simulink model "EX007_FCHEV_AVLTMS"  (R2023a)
settings: Solver=ode23tb  StartTime=0.0  StopTime=20e3  RelTol=1e-3
libraries: component_lib x76, slpidlib x7, simulink x1

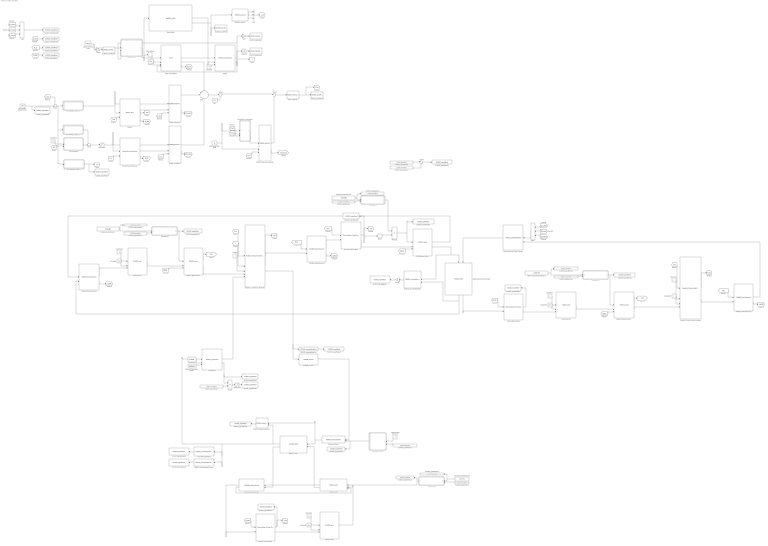
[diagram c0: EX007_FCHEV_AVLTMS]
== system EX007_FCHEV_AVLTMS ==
  Add : Sum  Inputs=+++
  Add1 : Sum  Inputs=+++
  Battery : component_lib/Battery Pack  SOC_0=0.5  Nx=120  Ny=180
  Battery Chiller : component_lib/Thermal Systems/RF0007_PHEX  N_ch=20  L=180e-3  B=65e-3  H=2e-3  t=0.3e-3  D_h=2.61e-3  N_nod=5
  Battery Thermal Mass : component_lib/Thermal Mass & Heat Transfer  n=100  d=10e-3  L=4  m=120 * 180 * 0.048  cp=1040  T_0=273 + 25
  Bus Voltage Control 1 : Subsystem
  "Bus Voltage Control 2 " : Subsystem
  Bus Voltage Control 3 : Subsystem
  Bus Voltage Reference [V] : Constant  Value=700
  Calculate Superheat1 : component_lib/Thermal Systems/RF0010_calculateSuperHeat
  Chassi : component_lib/Powertrain/PT0001_simpleVehicle  m=40e3  r_w=0.5  A_f=10  C_d=0.5  rho_air=1.225  c_r0=0.0060  c_r1=2.3e-7  gain=600  v0=75/3.6  x0=0
  Compressor : component_lib/Thermal Systems/RF0003_compressor  V_disp=0.00017  N_ref=2000
  Constant : Constant
  Constant1 : Constant  Value=0
  Constant10 : Constant
  Constant11 : Constant  Value=0
  Constant2 : Constant  Value=8
  Constant3 : Constant  Value=0.5
  Constant4 : Constant  Value=0.1
  Constant5 : Constant  Value=2e5
  Constant6 : Constant  Value=2e5
  Constant7 : Constant  Value=5
  Constant8 : Constant  Value=1.65e6
  Constant9 : Constant  Value=2e5
  Coolant Tank1 : component_lib/Thermal Systems/TH0013_tank  V=5e-3  T0=273.15 + 80
  Coolant Tank2 : component_lib/Thermal Systems/TH0013_tank  V=5e-3  T0=273.15 + 25
  Coolant Tank3 : component_lib/Thermal Systems/TH0013_tank  V=5e-3  T0=273.15 + 80
  DC/DC - Low level converter : component_lib/Electrochemistry/EL0008_dcdcConverter  eta_up=0.98  eta_down=0.98
  DC/DC Converter : component_lib/Electrochemistry/EL0008_dcdcConverter  eta_up=0.98  eta_down=0.98
  DC/DC Converter1 : component_lib/Electrochemistry/EL0008_dcdcConverter  eta_up=0.98  eta_down=0.98
  Divide : Product  Inputs=/*
  Expansion Valve : component_lib/Thermal Systems/RF0005_expansionValve  D=3*1.8e-3  p_min=100e3
  Fuel Cell Thermal Mass : component_lib/Thermal Mass & Heat Transfer  n=375*2*10  d=2e-3  L=50e-2  m=72  cp=420  T_0=273 + 80
  Gain : Gain  Gain=3.6
  Gain1 : Gain  Gain=3.6
  Gain4 : Gain  Gain=-1
  Gear selector : Relay  OnSwitchValue=22  OffSwitchValue=21.5  OnOutputValue=4  OffOutputValue=3
  Integrator : Integrator
  Liquid-Liquid Heat Exchanger : component_lib/Thermal Systems/TH0018_PHEX  N_ch=60  L=180e-3  B=65e-3  H=2e-3  t=0.3e-3  D_h=2.61e-3  N_nod=5
  Low Voltage Bus Level : Constant  Value=24
  Low level bus consumers : Subsystem
  MN0002_ambient : component_lib/Mission/MN0002_ambient  p_0=1.01e5  T_0=273 + 40  RH_0=0.05
  Motor Heat Transfer : component_lib/Thermal Mass & Heat Transfer  n=100*3  d=5e-3  L=30e-2  m=200  cp=420  T_0=273 + 20
  Motor Temperature Reference : Constant  Value=273+70
  Motor and Gearbox : component_lib/E-Axle  n=3  V_nom=700
  Mux : Mux  Inputs=3
  Nominal Compressor speed1 : Constant  Value=1500/60
  PHEX Bypass Valve : component_lib/Thermal Systems/TH0014_valve  d=10e-2  dr=5e-2  C_d=0.9
  Power Electronics Heat Transfer : component_lib/Thermal Systems/TH0015_totalHeatTransfer  SystemSampleTime=-1  VariantActivationTime=update diagram  Latency=0  AutoFrameSizeCalculation=off
  Product1 : Product
  RF0008_receiver : component_lib/Thermal Systems/RF0008_receiver  V=100e-3  h0=280e3  p0=1.5e6  p_gain=1e3
  RF0011_calculateSubCool : component_lib/Thermal Systems/RF0011_calculateSubCool
  RF0013_calculateHeatflow : component_lib/Thermal Systems/RF0013_calculateHeatflow
  RF0014_calculateVaporFraction : component_lib/Thermal Systems/RF0014_calculateVaporFraction
  Radiator & Condenser Assembly : component_lib/Radiator and Condenser Assembly
  Radiator Bypass Valve : component_lib/Thermal Systems/TH0014_valve  d=10e-2  dr=5e-2  C_d=0.9
  Radiator Bypass Valve1 : component_lib/Thermal Systems/TH0014_valve  d=10e-2  dr=5e-2  C_d=0.9
  Relay : Relay  OnSwitchValue=273.15 + 90  OffSwitchValue=273.15 + 85  OnOutputValue=0  OffOutputValue=1
  Road Profile : component_lib/Mission/MN0001_profile  profile=Munchen.mat  x0=0  N_lookahead=100
  SC0002_signalRead : component_lib/Data & Control/SC0002_signalRead  SigName=velocity
  SC0002_signalRead1 : component_lib/Data & Control/SC0002_signalRead  SigName=batteryGeneratedHeat
  SC0002_signalRead10 : component_lib/Data & Control/SC0002_signalRead  SigName=condenserSubcooling
  SC0002_signalRead11 : component_lib/Data & Control/SC0002_signalRead  SigName=chillerBypassValve
  SC0002_signalRead12 : component_lib/Data & Control/SC0002_signalRead  SigName=batteryTemperatureReference
  SC0002_signalRead13 : component_lib/Data & Control/SC0002_signalRead  SigName=evaporatorCooling
  SC0002_signalRead15 : component_lib/Data & Control/SC0002_signalRead  SigName=expansionValve
  SC0002_signalRead17 : component_lib/Data & Control/SC0002_signalRead  SigName=COOP
  SC0002_signalRead18 : component_lib/Data & Control/SC0002_signalRead  SigName=fuelCellTemperature
  SC0002_signalRead19 : component_lib/Data & Control/SC0002_signalRead  SigName=radiatorBypassValve
  SC0002_signalRead2 : component_lib/Data & Control/SC0002_signalRead  SigName=altitude
  SC0002_signalRead21 : component_lib/Data & Control/SC0002_signalRead  SigName=fuelCellTemperatureReference
  SC0002_signalRead22 : component_lib/Data & Control/SC0002_signalRead  SigName=batteryTemperature
  SC0002_signalRead23 : component_lib/Data & Control/SC0002_signalRead  SigName=motorGeneratedHeat
  SC0002_signalRead24 : component_lib/Data & Control/SC0002_signalRead  SigName=converterGeneratedHeat
  SC0002_signalRead25 : component_lib/Data & Control/SC0002_signalRead  SigName=motorTemperature
  SC0002_signalRead26 : component_lib/Data & Control/SC0002_signalRead  SigName=sideRadiatorBypassValve
  SC0002_signalRead27 : component_lib/Data & Control/SC0002_signalRead  SigName=motorTemperatureReference
  SC0002_signalRead28 : component_lib/Data & Control/SC0002_signalRead  SigName=PHEXBypassValve
  SC0002_signalRead3 : component_lib/Data & Control/SC0002_signalRead  SigName=velocityReference
  SC0002_signalRead30 : component_lib/Data & Control/SC0002_signalRead  SigName=PHEXCooling
  SC0002_signalRead31 : component_lib/Data & Control/SC0002_signalRead  SigName=fuelCellHighTemperatureReference
  SC0002_signalRead32 : component_lib/Data & Control/SC0002_signalRead  SigName=totalFuelCellCooling
  SC0002_signalRead38 : component_lib/Data & Control/SC0002_signalRead  SigName=evaporatorVaporFraction
  SC0002_signalRead4 : component_lib/Data & Control/SC0002_signalRead  SigName=busVoltage
  SC0002_signalRead40 : component_lib/Data & Control/SC0002_signalRead  SigName=evaporatorSuperheat
  SC0002_signalRead5 : component_lib/Data & Control/SC0002_signalRead  SigName=distance
  SC0002_signalRead6 : component_lib/Data & Control/SC0002_signalRead  SigName=busVoltageReference
  SC0002_signalRead7 : component_lib/Data & Control/SC0002_signalRead  SigName=burnoffCurrent
  SC0002_signalRead8 : component_lib/Data & Control/SC0002_signalRead  SigName=fuelCellGeneratedHeat
  SC0002_signalRead9 : component_lib/Data & Control/SC0002_signalRead  SigName=compressorPower
  SC0003_signalWrite1 : component_lib/Data & Control/SC0003_signalWrite  SigName=evaporatorCooling
  SC0003_signalWrite2 : component_lib/Data & Control/SC0003_signalWrite  SigName=evaporatorSuperheat
  SC0003_signalWrite3 : component_lib/Data & Control/SC0003_signalWrite  SigName=fuelCellTemperature
  SC0003_signalWrite4 : component_lib/Data & Control/SC0003_signalWrite  SigName=motorTemperature
  SC0003_signalWrite5 : component_lib/Data & Control/SC0003_signalWrite  SigName=fuelCellTemperature
  SC0003_signalWrite6 : component_lib/Data & Control/SC0003_signalWrite  SigName=radiatorCooling
  SC0003_signalWrite7 : component_lib/Data & Control/SC0003_signalWrite  SigName=PHEXCooling
  SC0003_signalWrite8 : component_lib/Data & Control/SC0003_signalWrite  SigName=batteryTemperature
  SOC-reference : Subsystem
  Saturation : Saturate  UpperLimit=600  LowerLimit=20
  Saturation1 : Saturate  UpperLimit=10  LowerLimit=0
  Simple Fuel Cell System : component_lib/Simple Fuel Cell System  n_st=2  n=375
  Single Air Stream Heat Exchanger : component_lib/Single Air Stream Heat Exchanger  HtH=1.1  StS=0.95
  Speed control : Subsystem
  Speed reference [m/s] : Constant  Value=75/3.6
  Subsystem1 : Subsystem
  Subsystem2 : Subsystem
  Subsystem3 : Subsystem
  Subsystem4 : Subsystem
  Sum : Sum  Inputs=-++
  Sum1 : Sum  Inputs=-+|
  Sum2 : Sum  Inputs=++|
  Sum3 : Sum  Inputs=|+-
  Sum4 : Sum  Inputs=|+-
  Sum8 : Sum  Inputs=|++
  Super Capacitor : component_lib/Electrochemistry/EL0010_superCapacitor  C=1  V_bus0=700
  Superheat Control : Subsystem
  Superheating Reference : Constant  Value=5
  TH0006_flowConfluence{,1..3} (4 alike) : component_lib/Thermal Systems/TH0006_flowConfluence  gain=0.01
  TH0014_valve : component_lib/Thermal Systems/TH0014_valve  d=10e-2  dr=5e-2  C_d=0.9
  TH0016_calculateHeatflow1 : component_lib/Thermal Systems/TH0016_calculateHeatflow
  Temperature Reference : Constant  Value=273+80
  Temperature Reference1 : Constant  Value=273+85
  Temperature Reference2 : Constant  Value=273+25
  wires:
  Motor and Gearbox/1 -> Chassi/1
  Chassi/2 -> Motor and Gearbox/4
  Road Profile/1 -> Chassi/2
  Chassi/1 -> [v], Gain/1, Speed control/2(v [m/s]), Road Profile/1, Gear selector/1, Integrator/1
  Speed reference [m/s]/1 -> Gain1/1, Speed control/1(v_ref [m/s])
  Speed control/1(Tq_sig [-]) -> Motor and Gearbox/1
  Gear selector/1 -> Motor and Gearbox/2
  Integrator/1 -> SC0002_signalRead5/1
  Gain/1 -> SC0002_signalRead/1
  Road Profile/2 -> SC0002_signalRead2/1, MN0002_ambient/1
  Gain1/1 -> SC0002_signalRead3/1
  Constant1/1 -> Chassi/3
  Battery/1 -> DC/DC Converter/2
  DC/DC Converter/1 -> Sum/2
  Motor and Gearbox/2 -> Sum/1
  Battery/2 -> [SOC]
  Bus Voltage Control 1/1(I_bat [-]) -> DC/DC Converter/1, Battery/1
  DC/DC Converter1/1 -> Sum/3
  Bus Voltage Reference [V]/1 -> Sum1/2, SC0002_signalRead6/1
  Constant3/1 -> SOC-reference/1(SOC_ref [-])
  [SOC] -> SOC-reference/2(SOC [-])
  Sum1/1 -> Bus Voltage Control 3/1(V_ref - V_bus [V]), "Bus Voltage Control 2 "/1(V_ref - V_bus [V]), Bus Voltage Control 1/1(V_ref - V_bus [V])
  Sum2/1 -> Saturation/1
  SOC-reference/1(I_fc_nom [A]) -> Sum2/2
  Sum/1 -> Sum3/1
  Bus Voltage Control 3/1(I_bf [A]) -> SC0002_signalRead7/1, [I_bf]
  [I_bf] -> Sum3/2
  MN0002_ambient/3 -> Mux/3
  MN0002_ambient/1 -> Mux/1
  MN0002_ambient/2 -> Mux/2
  Mux/1 -> [amb]
  Simple Fuel Cell System/1 -> DC/DC Converter1/2
  [T_fc] -> Simple Fuel Cell System/2
  Sum3/1 -> Sum4/1
  Saturation/1 -> DC/DC Converter1/1, Simple Fuel Cell System/1
  "Bus Voltage Control 2 "/1(I_fc+ [A]) -> Sum2/1
  Battery/3 -> [Q_bat]
  Simple Fuel Cell System/2 -> [Q_fc]
  [amb] -> Radiator & Condenser Assembly/1
  [v] -> Radiator & Condenser Assembly/2
  Constant/1 -> Radiator & Condenser Assembly/3
  RF0011_calculateSubCool/1 -> SC0002_signalRead10/1
  Divide/1 -> Saturation1/1
  Saturation1/1 -> SC0002_signalRead17/1
  Compressor/2 -> SC0002_signalRead9/1, Divide/1
  Superheat Control/1(EXV [-]) -> Expansion Valve/2, SC0002_signalRead15/1
  Superheating Reference/1 -> Superheat Control/1(T_ref [K])
  Super Capacitor/1 -> SC0002_signalRead4/1, [V_bus]
  [P_fan1] -> Low level bus consumers/2(P_1 [J/s])
  DC/DC - Low level converter/2 -> [Q_conv3]
  Low Voltage Bus Level/1 -> DC/DC - Low level converter/2, Low level bus consumers/1(V [V])
  DC/DC - Low level converter/1 -> Sum4/2
  Sum4/1 -> Super Capacitor/1
  Radiator & Condenser Assembly/1 -> [P_fan1]
  Motor and Gearbox/3 -> [Q_em]
  DC/DC Converter/2 -> [Q_conv1]
  DC/DC Converter1/2 -> [Q_conv2]
  [V_bus] -> Motor and Gearbox/3
  [V_bus] -> Sum1/1
  Fuel Cell Thermal Mass/1 -> Relay/1, [T_fc], SC0002_signalRead18/1
  [Q_fc] -> Fuel Cell Thermal Mass/1
  Temperature Reference/1 -> SC0002_signalRead21/1, Subsystem1/1(T_ref [K])
  Subsystem1/1(cv [-]) -> Radiator Bypass Valve/1, SC0002_signalRead19/1
  Radiator Bypass Valve/2 -> Radiator & Condenser Assembly/4
  SC0003_signalWrite3/1 -> Subsystem1/2(T_fc [K])
  Radiator & Condenser Assembly/2 -> TH0006_flowConfluence1/2
  TH0006_flowConfluence1/2 -> [split1]
  [split1] -> Radiator Bypass Valve/3
  Radiator Bypass Valve/1 -> [CL1]
  [CL1] -> TH0006_flowConfluence1/1
  Constant2/1 -> Coolant Tank1/1
  Constant5/1 -> Coolant Tank1/2
  Coolant Tank1/1 -> Radiator Bypass Valve/2
  [Q_bat] -> Battery Thermal Mass/1
  [Q_bat] -> SC0002_signalRead1/1
  [Q_fc] -> SC0002_signalRead8/1
  [T_bat] -> Battery/2
  Battery Thermal Mass/1 -> SC0002_signalRead22/1, [T_bat]
  [V_bus] -> DC/DC Converter/3
  [V_bus] -> DC/DC Converter1/3
  Battery Thermal Mass/2 -> Coolant Tank2/3
  Constant6/1 -> Coolant Tank2/2
  [V_bus] -> DC/DC - Low level converter/3
  Low level bus consumers/1(I [A]) -> DC/DC - Low level converter/1
  Constant4/1 -> Coolant Tank2/1
  SC0003_signalWrite1/1 -> Divide/2
  [Q_em] -> SC0002_signalRead23/1
  [Q_conv3] -> Add/3
  [Q_conv2] -> Add/2
  [Q_conv1] -> Add/1
  Add/1 -> SC0002_signalRead24/1
  Liquid-Liquid Heat Exchanger/2 -> Motor Heat Transfer/2
  [Q_conv3] -> Add1/3
  [Q_conv1] -> Add1/1
  [Q_conv2] -> Add1/2
  Add1/1 -> Power Electronics Heat Transfer/1
  [Q_em] -> Motor Heat Transfer/1
  Motor Heat Transfer/1 -> SC0002_signalRead25/1
  Motor Heat Transfer/2 -> Coolant Tank3/3
  Constant7/1 -> Coolant Tank3/1
  Constant9/1 -> Coolant Tank3/2
  SC0003_signalWrite4/1 -> Subsystem2/2(T_em [K])
  [split3] -> Radiator Bypass Valve1/3
  Subsystem2/1(cv [-]) -> Radiator Bypass Valve1/1, SC0002_signalRead26/1
  Motor Temperature Reference/1 -> SC0002_signalRead27/1, Subsystem2/1(T_ref [K])
  Constant10/1 -> Single Air Stream Heat Exchanger/3
  Constant11/1 -> Single Air Stream Heat Exchanger/2
  [amb] -> Single Air Stream Heat Exchanger/1
  [P_fan2] -> Low level bus consumers/3(P_2 [J/s])
  Single Air Stream Heat Exchanger/1 -> [P_fan2]
  Coolant Tank3/1 -> Radiator Bypass Valve1/2
  Radiator Bypass Valve1/2 -> Single Air Stream Heat Exchanger/4
  TH0006_flowConfluence2/2 -> [split3]
  [CL2] -> TH0006_flowConfluence2/1
  Single Air Stream Heat Exchanger/2 -> TH0006_flowConfluence2/2
  Radiator Bypass Valve1/1 -> [CL2]
  TH0006_flowConfluence2/1 -> Power Electronics Heat Transfer/2
  TH0006_flowConfluence1/1 -> Fuel Cell Thermal Mass/2
  Fuel Cell Thermal Mass/2 -> PHEX Bypass Valve/2
  PHEX Bypass Valve/2 -> TH0016_calculateHeatflow1/1, Liquid-Liquid Heat Exchanger/1
  Power Electronics Heat Transfer/1 -> Liquid-Liquid Heat Exchanger/2
  [split4] -> PHEX Bypass Valve/3
  TH0006_flowConfluence3/1 -> Coolant Tank1/3
  TH0006_flowConfluence3/2 -> [split4]
  PHEX Bypass Valve/1 -> TH0006_flowConfluence3/1
  Liquid-Liquid Heat Exchanger/1 -> TH0016_calculateHeatflow1/2, TH0006_flowConfluence3/2
  Relay/1 -> Product1/2
  SC0003_signalWrite5/1 -> Subsystem3/2(T_fc [K])
  Temperature Reference1/1 -> SC0002_signalRead31/1, Subsystem3/1(T_ref [K])
  Product1/1 -> SC0002_signalRead28/1, PHEX Bypass Valve/1
  Subsystem3/1(cv [-]) -> Product1/1
  TH0016_calculateHeatflow1/1 -> Gain4/1
  Gain4/1 -> SC0002_signalRead30/1
  SC0003_signalWrite6/1 -> Sum8/1
  SC0003_signalWrite7/1 -> Sum8/2
  Sum8/1 -> SC0002_signalRead32/1
  Nominal Compressor speed1/1 -> Compressor/3
  Compressor/1 -> Radiator & Condenser Assembly/5
  RF0014_calculateVaporFraction/1 -> SC0002_signalRead38/1
  SC0003_signalWrite2/1 -> Superheat Control/2(T_sup [K])
  Calculate Superheat1/1 -> SC0002_signalRead40/1
  Radiator & Condenser Assembly/3 -> RF0008_receiver/1, RF0011_calculateSubCool/1
  SC0003_signalWrite8/1 -> Subsystem4/2(T [K])
  Temperature Reference2/1 -> SC0002_signalRead12/1, Subsystem4/1(T_ref [K])
  Subsystem4/1(cv [-]) -> TH0014_valve/1, SC0002_signalRead11/1
  TH0014_valve/1 -> TH0006_flowConfluence/1
  TH0014_valve/2 -> Battery Chiller/2
  Battery Chiller/2 -> TH0006_flowConfluence/2
  TH0006_flowConfluence/1 -> Battery Thermal Mass/2
  TH0006_flowConfluence/2 -> TH0014_valve/3
  Coolant Tank2/1 -> TH0014_valve/2
  Expansion Valve/1 -> RF0013_calculateHeatflow/1, Battery Chiller/1
  RF0013_calculateHeatflow/1 -> SC0002_signalRead13/1
  Battery Chiller/1 -> RF0013_calculateHeatflow/2, RF0014_calculateVaporFraction/1, Calculate Superheat1/1, Compressor/1
  RF0008_receiver/1 -> Expansion Valve/1
  Constant8/1 -> Compressor/2

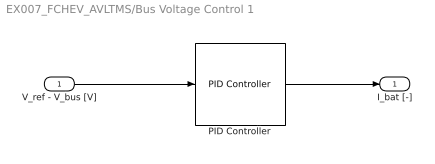
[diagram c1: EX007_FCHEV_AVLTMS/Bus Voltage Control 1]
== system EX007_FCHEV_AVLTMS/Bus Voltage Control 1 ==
  V_ref - V_bus [V] : Inport
  PID Controller : slpidlib/PID Controller  Controller=PID  Form=Parallel  TimeDomain=Continuous-time  UseExternalTs=off  SampleTime=-1  IntegratorMethod=Forward Euler  FilterMethod=Forward Euler  ControllerParametersSource=internal  P=1e2  I=1  UseKiTs=off  D=0  N=100  UseFilter=on  TunerSelectOption=Transfer Function Based (PID Tuner App)  ZeroCross=off  InitialConditionSource=internal  InitialConditionForIntegrator=0  InitialConditionForFilter=0  DifferentiatorICPrevScaledInput=0  ExternalReset=none  TrackingMode=off  Kt=1  LimitOutput=on  SatLimitsSource=internal  UpperSaturationLimit=600  LowerSaturationLimit=-350  LinearizeAsGain=on  AntiWindupMode=clamping  Kb=1  LimitIntegrator=off  UpperIntegratorSaturationLimit=inf  LowerIntegratorSaturationLimit=-inf  POutMin=[]  POutMax=[]  IOutMin=[]  IOutMax=[]  DOutMin=[]  DOutMax=[]  NOutMin=[]  NOutMax=[]  SumOutMin=[]  SumOutMax=[]  SaturationOutMin=[]  SaturationOutMax=[]  PParamMin=[]  PParamMax=[]  IParamMin=[]  IParamMax=[]  DParamMin=[]  DParamMax=[]  NParamMin=[]  NParamMax=[]  KbParamMin=[]  KbParamMax=[]  KtParamMin=[]  KtParamMax=[]  KbOutMin=[]  KbOutMax=[]  KtOutMin=[]  KtOutMax=[]  IntegratorOutMin=[]  IntegratorOutMax=[]  FilterOutMin=[]  FilterOutMax=[]  SumI1OutMin=[]  SumI1OutMax=[]  SumI2OutMin=[]  SumI2OutMax=[]  SumI3OutMin=[]  SumI3OutMax=[]  SumI4OutMin=[]  SumI4OutMax=[]  SumDOutMin=[]  SumDOutMax=[]  DifferentiatorOutMin=[]  DifferentiatorOutMax=[]  FilterDiffOutCoefMin=[]  FilterDiffOutCoefMax=[]  ReciprocalOutMin=[]  ReciprocalOutMax=[]  SumDenOutMin=[]  SumDenOutMax=[]  SumNumOutMin=[]  SumNumOutMax=[]  DivideOutMin=[]  DivideOutMax=[]  UdiffTsProdOutMin=[]  UdiffTsProdOutMax=[]  NTsProdOutMin=[]  NTsProdOutMax=[]  UintegralTsProdOutMin=[]  UintegralTsProdOutMax=[]  UngainTsProdOutMin=[]  UngainTsProdOutMax=[]  ClampingZeroOutDataTypeStr=Inherit: Inherit via back propagation  ClampingZeroOutMin=[]  ClampingZeroOutMax=[]  FilterDenConstantOutDataTypeStr=Inherit: Inherit via back propagation  FilterDenConstantOutMin=[]  FilterDenConstantOutMax=[]  PCopyOutDataTypeStr=Inherit: Inherit via back propagation  PCopyOutMin=[]  PCopyOutMax=[]  NCopyOutDataTypeStr=Inherit: Inherit via back propagation  NCopyOutMin=[]  NCopyOutMax=[]  IntegratorContinuousStateAttributes=''  IntegratorStateMustResolveToSignalObject=off  IntegratorRTWStateStorageClass=Auto  FilterContinuousStateAttributes=''  FilterStateMustResolveToSignalObject=off  FilterRTWStateStorageClass=Auto  ParallelPVariant=InternalParameters  IdealPVariant=Disabled  IVariant=InternalParameters  DVariant=InternalParameters  IntegratorVariant=Continuous  SatVariant=Enabled  AWVariant=ContClampingParallel  PCopyVariant=Disabled  TRVariant=Disabled  FdbkBlocksVariant=Forward  IdealPFdbkVariant=Disabled  SatFdbkVariant=Disabled  DerivativeFilterVariant=ContFilter  NVariant=InternalParameters  NCopyVariant=Disabled  FilterICVariant=InternalICsFilter  IntegratorICVariant=InternalICs  ExternalResetVariant=Disabled  TRSumVariant=Passthrough  SumFdbkVariant=Disabled  SumVariant=Sum_PID  TsampFilterVariant=InternalTs  TsampNgainVariant=Passthrough  TsampIntegralVariant=Disabled_SignalSpec  ExternalSaturationOutDataTypeStr=Inherit: Same as second input
  I_bat [-] : Outport
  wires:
  PID Controller/1 -> I_bat [-]/1
  V_ref - V_bus [V]/1 -> PID Controller/1

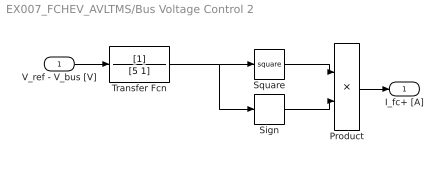
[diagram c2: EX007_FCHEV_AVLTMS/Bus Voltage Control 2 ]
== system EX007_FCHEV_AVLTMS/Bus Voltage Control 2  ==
  V_ref - V_bus [V] : Inport
  Product : Product
  Sign : Signum
  Square : Math  Operator=square
  Transfer Fcn : TransferFcn  Denominator=[5 1]
  I_fc+ [A] : Outport
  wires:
  Sign/1 -> Product/2
  Transfer Fcn/1 -> Sign/1, Square/1
  Square/1 -> Product/1
  V_ref - V_bus [V]/1 -> Transfer Fcn/1
  Product/1 -> I_fc+ [A]/1

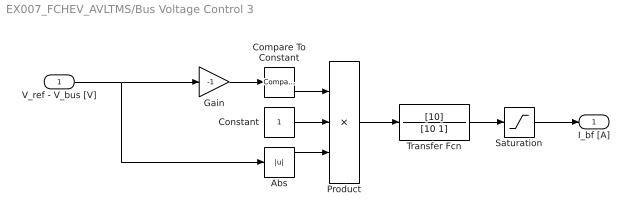
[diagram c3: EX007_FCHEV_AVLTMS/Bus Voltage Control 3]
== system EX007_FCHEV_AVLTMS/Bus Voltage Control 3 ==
  V_ref - V_bus [V] : Inport
  Abs : Abs
  Compare To Constant : simulink/Logic and Bit Operations/Compare To Constant  relop=>=  const=30  OutDataTypeStr=boolean
  Constant : Constant
  Gain : Gain  Gain=-1
  Product : Product  Inputs=3
  Saturation : Saturate  UpperLimit=1000  LowerLimit=0
  Transfer Fcn : TransferFcn  Numerator=[10]  Denominator=[10 1]
  I_bf [A] : Outport
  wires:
  Gain/1 -> Compare To Constant/1
  Transfer Fcn/1 -> Saturation/1
  Compare To Constant/1 -> Product/1
  Product/1 -> Transfer Fcn/1
  V_ref - V_bus [V]/1 -> Abs/1, Gain/1
  Abs/1 -> Product/3
  Constant/1 -> Product/2
  Saturation/1 -> I_bf [A]/1

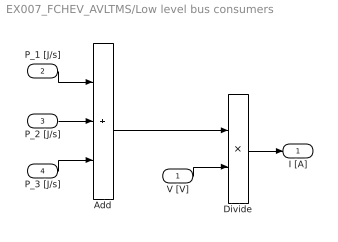
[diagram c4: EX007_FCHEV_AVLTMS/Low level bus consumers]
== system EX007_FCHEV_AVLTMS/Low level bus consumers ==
  V [V] : Inport
  P_1 [J/s] : Inport  Port=2
  P_2 [J/s] : Inport  Port=3
  P_3 [J/s] : Inport  Port=4
  Add : Sum  Inputs=+++
  Divide : Product  Inputs=*/
  I [A] : Outport
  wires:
  Add/1 -> Divide/1
  P_1 [J/s]/1 -> Add/1
  V [V]/1 -> Divide/2
  P_3 [J/s]/1 -> Add/3
  P_2 [J/s]/1 -> Add/2
  Divide/1 -> I [A]/1

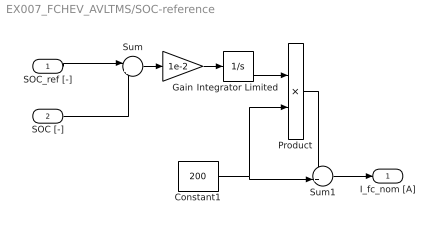
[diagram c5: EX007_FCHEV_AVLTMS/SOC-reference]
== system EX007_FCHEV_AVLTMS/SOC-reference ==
  SOC_ref [-] : Inport
  SOC [-] : Inport  Port=2
  Constant1 : Constant  Value=200
  Gain : Gain  Gain=1e-2
  Integrator Limited : Integrator  LimitOutput=on  UpperSaturationLimit=1  LowerSaturationLimit=-1
  Product : Product
  Sum : Sum  Inputs=|+-
  Sum1 : Sum  Inputs=++|
  I_fc_nom [A] : Outport
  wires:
  Product/1 -> Sum1/1
  Integrator Limited/1 -> Product/1
  Sum1/1 -> I_fc_nom [A]/1
  Constant1/1 -> Sum1/2, Product/2
  Sum/1 -> Gain/1
  SOC [-]/1 -> Sum/2
  Gain/1 -> Integrator Limited/1
  SOC_ref [-]/1 -> Sum/1

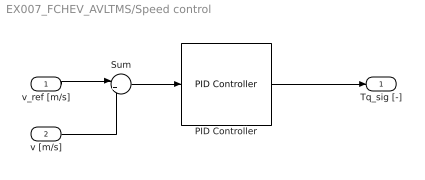
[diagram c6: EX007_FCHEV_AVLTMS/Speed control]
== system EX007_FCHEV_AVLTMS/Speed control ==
  v_ref [m/s] : Inport
  v [m/s] : Inport  Port=2
  PID Controller : slpidlib/PID Controller  Controller=PID  Form=Parallel  TimeDomain=Continuous-time  UseExternalTs=off  SampleTime=-1  IntegratorMethod=Forward Euler  FilterMethod=Forward Euler  ControllerParametersSource=internal  P=10  I=1e-1  UseKiTs=off  D=0  N=100  UseFilter=on  TunerSelectOption=Transfer Function Based (PID Tuner App)  ZeroCross=off  InitialConditionSource=internal  InitialConditionForIntegrator=0  InitialConditionForFilter=0  DifferentiatorICPrevScaledInput=0  ExternalReset=none  TrackingMode=off  Kt=1  LimitOutput=on  SatLimitsSource=internal  UpperSaturationLimit=1  LowerSaturationLimit=-1  LinearizeAsGain=on  AntiWindupMode=clamping  Kb=1  LimitIntegrator=off  UpperIntegratorSaturationLimit=inf  LowerIntegratorSaturationLimit=-inf  POutMin=[]  POutMax=[]  IOutMin=[]  IOutMax=[]  DOutMin=[]  DOutMax=[]  NOutMin=[]  NOutMax=[]  SumOutMin=[]  SumOutMax=[]  SaturationOutMin=[]  SaturationOutMax=[]  PParamMin=[]  PParamMax=[]  IParamMin=[]  IParamMax=[]  DParamMin=[]  DParamMax=[]  NParamMin=[]  NParamMax=[]  KbParamMin=[]  KbParamMax=[]  KtParamMin=[]  KtParamMax=[]  KbOutMin=[]  KbOutMax=[]  KtOutMin=[]  KtOutMax=[]  IntegratorOutMin=[]  IntegratorOutMax=[]  FilterOutMin=[]  FilterOutMax=[]  SumI1OutMin=[]  SumI1OutMax=[]  SumI2OutMin=[]  SumI2OutMax=[]  SumI3OutMin=[]  SumI3OutMax=[]  SumI4OutMin=[]  SumI4OutMax=[]  SumDOutMin=[]  SumDOutMax=[]  DifferentiatorOutMin=[]  DifferentiatorOutMax=[]  FilterDiffOutCoefMin=[]  FilterDiffOutCoefMax=[]  ReciprocalOutMin=[]  ReciprocalOutMax=[]  SumDenOutMin=[]  SumDenOutMax=[]  SumNumOutMin=[]  SumNumOutMax=[]  DivideOutMin=[]  DivideOutMax=[]  UdiffTsProdOutMin=[]  UdiffTsProdOutMax=[]  NTsProdOutMin=[]  NTsProdOutMax=[]  UintegralTsProdOutMin=[]  UintegralTsProdOutMax=[]  UngainTsProdOutMin=[]  UngainTsProdOutMax=[]  ClampingZeroOutDataTypeStr=Inherit: Inherit via back propagation  ClampingZeroOutMin=[]  ClampingZeroOutMax=[]  FilterDenConstantOutDataTypeStr=Inherit: Inherit via back propagation  FilterDenConstantOutMin=[]  FilterDenConstantOutMax=[]  PCopyOutDataTypeStr=Inherit: Inherit via back propagation  PCopyOutMin=[]  PCopyOutMax=[]  NCopyOutDataTypeStr=Inherit: Inherit via back propagation  NCopyOutMin=[]  NCopyOutMax=[]  IntegratorContinuousStateAttributes=''  IntegratorStateMustResolveToSignalObject=off  IntegratorRTWStateStorageClass=Auto  FilterContinuousStateAttributes=''  FilterStateMustResolveToSignalObject=off  FilterRTWStateStorageClass=Auto  ParallelPVariant=InternalParameters  IdealPVariant=Disabled  IVariant=InternalParameters  DVariant=InternalParameters  IntegratorVariant=Continuous  SatVariant=Enabled  AWVariant=ContClampingParallel  PCopyVariant=Disabled  TRVariant=Disabled  FdbkBlocksVariant=Forward  IdealPFdbkVariant=Disabled  SatFdbkVariant=Disabled  DerivativeFilterVariant=ContFilter  NVariant=InternalParameters  NCopyVariant=Disabled  FilterICVariant=InternalICsFilter  IntegratorICVariant=InternalICs  ExternalResetVariant=Disabled  TRSumVariant=Passthrough  SumFdbkVariant=Disabled  SumVariant=Sum_PID  TsampFilterVariant=InternalTs  TsampNgainVariant=Passthrough  TsampIntegralVariant=Disabled_SignalSpec  ExternalSaturationOutDataTypeStr=Inherit: Same as second input
  Sum : Sum  Inputs=|+-
  Tq_sig [-] : Outport
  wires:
  PID Controller/1 -> Tq_sig [-]/1
  Sum/1 -> PID Controller/1
  v_ref [m/s]/1 -> Sum/1
  v [m/s]/1 -> Sum/2

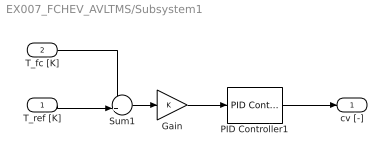
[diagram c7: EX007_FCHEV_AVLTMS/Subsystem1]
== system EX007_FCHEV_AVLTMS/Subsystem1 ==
  T_ref [K] : Inport
  T_fc [K] : Inport  Port=2
  Gain : Gain
  PID Controller1 : slpidlib/PID Controller  Controller=PI  Form=Parallel  TimeDomain=Continuous-time  UseExternalTs=off  SampleTime=-1  IntegratorMethod=Forward Euler  FilterMethod=Forward Euler  ControllerParametersSource=internal  P=1e-1  I=1e-3  UseKiTs=off  D=0  N=100  UseFilter=on  TunerSelectOption=Transfer Function Based (PID Tuner App)  ZeroCross=off  InitialConditionSource=internal  InitialConditionForIntegrator=0.5  InitialConditionForFilter=0.5  DifferentiatorICPrevScaledInput=0  ExternalReset=none  TrackingMode=off  Kt=1  LimitOutput=on  SatLimitsSource=internal  UpperSaturationLimit=1  LowerSaturationLimit=0  LinearizeAsGain=on  AntiWindupMode=clamping  Kb=1  LimitIntegrator=off  UpperIntegratorSaturationLimit=inf  LowerIntegratorSaturationLimit=-inf  POutMin=[]  POutMax=[]  IOutMin=[]  IOutMax=[]  DOutMin=[]  DOutMax=[]  NOutMin=[]  NOutMax=[]  SumOutMin=[]  SumOutMax=[]  SaturationOutMin=[]  SaturationOutMax=[]  PParamMin=[]  PParamMax=[]  IParamMin=[]  IParamMax=[]  DParamMin=[]  DParamMax=[]  NParamMin=[]  NParamMax=[]  KbParamMin=[]  KbParamMax=[]  KtParamMin=[]  KtParamMax=[]  KbOutMin=[]  KbOutMax=[]  KtOutMin=[]  KtOutMax=[]  IntegratorOutMin=[]  IntegratorOutMax=[]  FilterOutMin=[]  FilterOutMax=[]  SumI1OutMin=[]  SumI1OutMax=[]  SumI2OutMin=[]  SumI2OutMax=[]  SumI3OutMin=[]  SumI3OutMax=[]  SumI4OutMin=[]  SumI4OutMax=[]  SumDOutMin=[]  SumDOutMax=[]  DifferentiatorOutMin=[]  DifferentiatorOutMax=[]  FilterDiffOutCoefMin=[]  FilterDiffOutCoefMax=[]  ReciprocalOutMin=[]  ReciprocalOutMax=[]  SumDenOutMin=[]  SumDenOutMax=[]  SumNumOutMin=[]  SumNumOutMax=[]  DivideOutMin=[]  DivideOutMax=[]  UdiffTsProdOutMin=[]  UdiffTsProdOutMax=[]  NTsProdOutMin=[]  NTsProdOutMax=[]  UintegralTsProdOutMin=[]  UintegralTsProdOutMax=[]  UngainTsProdOutMin=[]  UngainTsProdOutMax=[]  ClampingZeroOutDataTypeStr=Inherit: Inherit via back propagation  ClampingZeroOutMin=[]  ClampingZeroOutMax=[]  FilterDenConstantOutDataTypeStr=Inherit: Inherit via back propagation  FilterDenConstantOutMin=[]  FilterDenConstantOutMax=[]  PCopyOutDataTypeStr=Inherit: Inherit via back propagation  PCopyOutMin=[]  PCopyOutMax=[]  NCopyOutDataTypeStr=Inherit: Inherit via back propagation  NCopyOutMin=[]  NCopyOutMax=[]  IntegratorContinuousStateAttributes=''  IntegratorStateMustResolveToSignalObject=off  IntegratorRTWStateStorageClass=Auto  FilterContinuousStateAttributes=''  FilterStateMustResolveToSignalObject=off  FilterRTWStateStorageClass=Auto  ParallelPVariant=InternalParameters  IdealPVariant=Disabled  IVariant=InternalParameters  DVariant=Disabled  IntegratorVariant=Continuous  SatVariant=Enabled  AWVariant=ContClampingParallel  PCopyVariant=Disabled  TRVariant=Disabled  FdbkBlocksVariant=Forward  IdealPFdbkVariant=Disabled  SatFdbkVariant=Disabled  DerivativeFilterVariant=Disabled  NVariant=Disabled  NCopyVariant=Disabled_SignalSpec  FilterICVariant=Disabled  IntegratorICVariant=InternalICs  ExternalResetVariant=Disabled  TRSumVariant=Passthrough  SumFdbkVariant=Disabled  SumVariant=Sum_PI  TsampFilterVariant=InternalTs  TsampNgainVariant=Passthrough  TsampIntegralVariant=Disabled_SignalSpec  ExternalSaturationOutDataTypeStr=Inherit: Same as second input
  Sum1 : Sum  Inputs=-+|
  cv [-] : Outport
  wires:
  T_fc [K]/1 -> Sum1/1
  Gain/1 -> PID Controller1/1
  Sum1/1 -> Gain/1
  PID Controller1/1 -> cv [-]/1
  T_ref [K]/1 -> Sum1/2

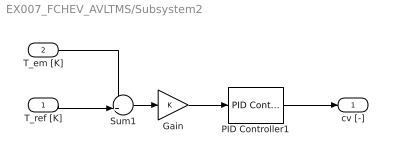
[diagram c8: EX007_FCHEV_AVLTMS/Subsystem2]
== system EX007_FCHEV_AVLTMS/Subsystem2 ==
  T_ref [K] : Inport
  T_em [K] : Inport  Port=2
  Gain : Gain
  PID Controller1 : slpidlib/PID Controller  Controller=PI  Form=Parallel  TimeDomain=Continuous-time  UseExternalTs=off  SampleTime=-1  IntegratorMethod=Forward Euler  FilterMethod=Forward Euler  ControllerParametersSource=internal  P=1e-1  I=1e-3  UseKiTs=off  D=0  N=100  UseFilter=on  TunerSelectOption=Transfer Function Based (PID Tuner App)  ZeroCross=off  InitialConditionSource=internal  InitialConditionForIntegrator=0.5  InitialConditionForFilter=0.5  DifferentiatorICPrevScaledInput=0  ExternalReset=none  TrackingMode=off  Kt=1  LimitOutput=on  SatLimitsSource=internal  UpperSaturationLimit=0.95  LowerSaturationLimit=0.05  LinearizeAsGain=on  AntiWindupMode=back-calculation  Kb=1  LimitIntegrator=off  UpperIntegratorSaturationLimit=inf  LowerIntegratorSaturationLimit=-inf  POutMin=[]  POutMax=[]  IOutMin=[]  IOutMax=[]  DOutMin=[]  DOutMax=[]  NOutMin=[]  NOutMax=[]  SumOutMin=[]  SumOutMax=[]  SaturationOutMin=[]  SaturationOutMax=[]  PParamMin=[]  PParamMax=[]  IParamMin=[]  IParamMax=[]  DParamMin=[]  DParamMax=[]  NParamMin=[]  NParamMax=[]  KbParamMin=[]  KbParamMax=[]  KtParamMin=[]  KtParamMax=[]  KbOutMin=[]  KbOutMax=[]  KtOutMin=[]  KtOutMax=[]  IntegratorOutMin=[]  IntegratorOutMax=[]  FilterOutMin=[]  FilterOutMax=[]  SumI1OutMin=[]  SumI1OutMax=[]  SumI2OutMin=[]  SumI2OutMax=[]  SumI3OutMin=[]  SumI3OutMax=[]  SumI4OutMin=[]  SumI4OutMax=[]  SumDOutMin=[]  SumDOutMax=[]  DifferentiatorOutMin=[]  DifferentiatorOutMax=[]  FilterDiffOutCoefMin=[]  FilterDiffOutCoefMax=[]  ReciprocalOutMin=[]  ReciprocalOutMax=[]  SumDenOutMin=[]  SumDenOutMax=[]  SumNumOutMin=[]  SumNumOutMax=[]  DivideOutMin=[]  DivideOutMax=[]  UdiffTsProdOutMin=[]  UdiffTsProdOutMax=[]  NTsProdOutMin=[]  NTsProdOutMax=[]  UintegralTsProdOutMin=[]  UintegralTsProdOutMax=[]  UngainTsProdOutMin=[]  UngainTsProdOutMax=[]  ClampingZeroOutDataTypeStr=Inherit: Inherit via back propagation  ClampingZeroOutMin=[]  ClampingZeroOutMax=[]  FilterDenConstantOutDataTypeStr=Inherit: Inherit via back propagation  FilterDenConstantOutMin=[]  FilterDenConstantOutMax=[]  PCopyOutDataTypeStr=Inherit: Inherit via back propagation  PCopyOutMin=[]  PCopyOutMax=[]  NCopyOutDataTypeStr=Inherit: Inherit via back propagation  NCopyOutMin=[]  NCopyOutMax=[]  IntegratorContinuousStateAttributes=''  IntegratorStateMustResolveToSignalObject=off  IntegratorRTWStateStorageClass=Auto  FilterContinuousStateAttributes=''  FilterStateMustResolveToSignalObject=off  FilterRTWStateStorageClass=Auto  ParallelPVariant=InternalParameters  IdealPVariant=Disabled  IVariant=InternalParameters  DVariant=Disabled  IntegratorVariant=Continuous  SatVariant=Enabled  AWVariant=BackCalculation  PCopyVariant=Disabled  TRVariant=Disabled  FdbkBlocksVariant=Forward  IdealPFdbkVariant=Disabled  SatFdbkVariant=Disabled  DerivativeFilterVariant=Disabled  NVariant=Disabled  NCopyVariant=Disabled_SignalSpec  FilterICVariant=Disabled  IntegratorICVariant=InternalICs  ExternalResetVariant=Disabled  TRSumVariant=Passthrough  SumFdbkVariant=Disabled  SumVariant=Sum_PI  TsampFilterVariant=InternalTs  TsampNgainVariant=Passthrough  TsampIntegralVariant=Disabled_SignalSpec  ExternalSaturationOutDataTypeStr=Inherit: Same as second input
  Sum1 : Sum  Inputs=-+|
  cv [-] : Outport
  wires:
  T_em [K]/1 -> Sum1/1
  Gain/1 -> PID Controller1/1
  Sum1/1 -> Gain/1
  PID Controller1/1 -> cv [-]/1
  T_ref [K]/1 -> Sum1/2

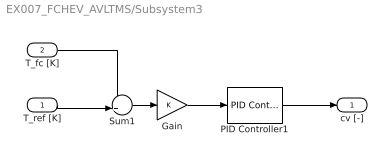
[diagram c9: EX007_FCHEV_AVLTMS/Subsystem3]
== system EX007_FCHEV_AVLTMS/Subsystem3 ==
  T_ref [K] : Inport
  T_fc [K] : Inport  Port=2
  Gain : Gain
  PID Controller1 : slpidlib/PID Controller  Controller=PI  Form=Parallel  TimeDomain=Continuous-time  UseExternalTs=off  SampleTime=-1  IntegratorMethod=Forward Euler  FilterMethod=Forward Euler  ControllerParametersSource=internal  P=1e-1  I=1e-3  UseKiTs=off  D=0  N=100  UseFilter=on  TunerSelectOption=Transfer Function Based (PID Tuner App)  ZeroCross=off  InitialConditionSource=internal  InitialConditionForIntegrator=0.5  InitialConditionForFilter=0.5  DifferentiatorICPrevScaledInput=0  ExternalReset=none  TrackingMode=off  Kt=1  LimitOutput=on  SatLimitsSource=internal  UpperSaturationLimit=1  LowerSaturationLimit=0  LinearizeAsGain=on  AntiWindupMode=back-calculation  Kb=1  LimitIntegrator=off  UpperIntegratorSaturationLimit=inf  LowerIntegratorSaturationLimit=-inf  POutMin=[]  POutMax=[]  IOutMin=[]  IOutMax=[]  DOutMin=[]  DOutMax=[]  NOutMin=[]  NOutMax=[]  SumOutMin=[]  SumOutMax=[]  SaturationOutMin=[]  SaturationOutMax=[]  PParamMin=[]  PParamMax=[]  IParamMin=[]  IParamMax=[]  DParamMin=[]  DParamMax=[]  NParamMin=[]  NParamMax=[]  KbParamMin=[]  KbParamMax=[]  KtParamMin=[]  KtParamMax=[]  KbOutMin=[]  KbOutMax=[]  KtOutMin=[]  KtOutMax=[]  IntegratorOutMin=[]  IntegratorOutMax=[]  FilterOutMin=[]  FilterOutMax=[]  SumI1OutMin=[]  SumI1OutMax=[]  SumI2OutMin=[]  SumI2OutMax=[]  SumI3OutMin=[]  SumI3OutMax=[]  SumI4OutMin=[]  SumI4OutMax=[]  SumDOutMin=[]  SumDOutMax=[]  DifferentiatorOutMin=[]  DifferentiatorOutMax=[]  FilterDiffOutCoefMin=[]  FilterDiffOutCoefMax=[]  ReciprocalOutMin=[]  ReciprocalOutMax=[]  SumDenOutMin=[]  SumDenOutMax=[]  SumNumOutMin=[]  SumNumOutMax=[]  DivideOutMin=[]  DivideOutMax=[]  UdiffTsProdOutMin=[]  UdiffTsProdOutMax=[]  NTsProdOutMin=[]  NTsProdOutMax=[]  UintegralTsProdOutMin=[]  UintegralTsProdOutMax=[]  UngainTsProdOutMin=[]  UngainTsProdOutMax=[]  ClampingZeroOutDataTypeStr=Inherit: Inherit via back propagation  ClampingZeroOutMin=[]  ClampingZeroOutMax=[]  FilterDenConstantOutDataTypeStr=Inherit: Inherit via back propagation  FilterDenConstantOutMin=[]  FilterDenConstantOutMax=[]  PCopyOutDataTypeStr=Inherit: Inherit via back propagation  PCopyOutMin=[]  PCopyOutMax=[]  NCopyOutDataTypeStr=Inherit: Inherit via back propagation  NCopyOutMin=[]  NCopyOutMax=[]  IntegratorContinuousStateAttributes=''  IntegratorStateMustResolveToSignalObject=off  IntegratorRTWStateStorageClass=Auto  FilterContinuousStateAttributes=''  FilterStateMustResolveToSignalObject=off  FilterRTWStateStorageClass=Auto  ParallelPVariant=InternalParameters  IdealPVariant=Disabled  IVariant=InternalParameters  DVariant=Disabled  IntegratorVariant=Continuous  SatVariant=Enabled  AWVariant=BackCalculation  PCopyVariant=Disabled  TRVariant=Disabled  FdbkBlocksVariant=Forward  IdealPFdbkVariant=Disabled  SatFdbkVariant=Disabled  DerivativeFilterVariant=Disabled  NVariant=Disabled  NCopyVariant=Disabled_SignalSpec  FilterICVariant=Disabled  IntegratorICVariant=InternalICs  ExternalResetVariant=Disabled  TRSumVariant=Passthrough  SumFdbkVariant=Disabled  SumVariant=Sum_PI  TsampFilterVariant=InternalTs  TsampNgainVariant=Passthrough  TsampIntegralVariant=Disabled_SignalSpec  ExternalSaturationOutDataTypeStr=Inherit: Same as second input
  Sum1 : Sum  Inputs=-+|
  cv [-] : Outport
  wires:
  T_fc [K]/1 -> Sum1/1
  Gain/1 -> PID Controller1/1
  Sum1/1 -> Gain/1
  PID Controller1/1 -> cv [-]/1
  T_ref [K]/1 -> Sum1/2

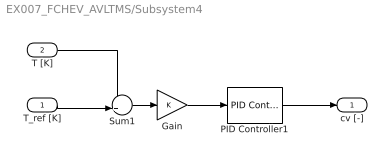
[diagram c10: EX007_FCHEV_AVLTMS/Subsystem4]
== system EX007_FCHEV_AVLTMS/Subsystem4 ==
  T_ref [K] : Inport
  T [K] : Inport  Port=2
  Gain : Gain
  PID Controller1 : slpidlib/PID Controller  Controller=PI  Form=Parallel  TimeDomain=Continuous-time  UseExternalTs=off  SampleTime=-1  IntegratorMethod=Forward Euler  FilterMethod=Forward Euler  ControllerParametersSource=internal  P=1e-1  I=1e-3  UseKiTs=off  D=0  N=100  UseFilter=on  TunerSelectOption=Transfer Function Based (PID Tuner App)  ZeroCross=off  InitialConditionSource=internal  InitialConditionForIntegrator=0.5  InitialConditionForFilter=0.5  DifferentiatorICPrevScaledInput=0  ExternalReset=none  TrackingMode=off  Kt=1  LimitOutput=on  SatLimitsSource=internal  UpperSaturationLimit=1  LowerSaturationLimit=0  LinearizeAsGain=on  AntiWindupMode=back-calculation  Kb=1  LimitIntegrator=off  UpperIntegratorSaturationLimit=inf  LowerIntegratorSaturationLimit=-inf  POutMin=[]  POutMax=[]  IOutMin=[]  IOutMax=[]  DOutMin=[]  DOutMax=[]  NOutMin=[]  NOutMax=[]  SumOutMin=[]  SumOutMax=[]  SaturationOutMin=[]  SaturationOutMax=[]  PParamMin=[]  PParamMax=[]  IParamMin=[]  IParamMax=[]  DParamMin=[]  DParamMax=[]  NParamMin=[]  NParamMax=[]  KbParamMin=[]  KbParamMax=[]  KtParamMin=[]  KtParamMax=[]  KbOutMin=[]  KbOutMax=[]  KtOutMin=[]  KtOutMax=[]  IntegratorOutMin=[]  IntegratorOutMax=[]  FilterOutMin=[]  FilterOutMax=[]  SumI1OutMin=[]  SumI1OutMax=[]  SumI2OutMin=[]  SumI2OutMax=[]  SumI3OutMin=[]  SumI3OutMax=[]  SumI4OutMin=[]  SumI4OutMax=[]  SumDOutMin=[]  SumDOutMax=[]  DifferentiatorOutMin=[]  DifferentiatorOutMax=[]  FilterDiffOutCoefMin=[]  FilterDiffOutCoefMax=[]  ReciprocalOutMin=[]  ReciprocalOutMax=[]  SumDenOutMin=[]  SumDenOutMax=[]  SumNumOutMin=[]  SumNumOutMax=[]  DivideOutMin=[]  DivideOutMax=[]  UdiffTsProdOutMin=[]  UdiffTsProdOutMax=[]  NTsProdOutMin=[]  NTsProdOutMax=[]  UintegralTsProdOutMin=[]  UintegralTsProdOutMax=[]  UngainTsProdOutMin=[]  UngainTsProdOutMax=[]  ClampingZeroOutDataTypeStr=Inherit: Inherit via back propagation  ClampingZeroOutMin=[]  ClampingZeroOutMax=[]  FilterDenConstantOutDataTypeStr=Inherit: Inherit via back propagation  FilterDenConstantOutMin=[]  FilterDenConstantOutMax=[]  PCopyOutDataTypeStr=Inherit: Inherit via back propagation  PCopyOutMin=[]  PCopyOutMax=[]  NCopyOutDataTypeStr=Inherit: Inherit via back propagation  NCopyOutMin=[]  NCopyOutMax=[]  IntegratorContinuousStateAttributes=''  IntegratorStateMustResolveToSignalObject=off  IntegratorRTWStateStorageClass=Auto  FilterContinuousStateAttributes=''  FilterStateMustResolveToSignalObject=off  FilterRTWStateStorageClass=Auto  ParallelPVariant=InternalParameters  IdealPVariant=Disabled  IVariant=InternalParameters  DVariant=Disabled  IntegratorVariant=Continuous  SatVariant=Enabled  AWVariant=BackCalculation  PCopyVariant=Disabled  TRVariant=Disabled  FdbkBlocksVariant=Forward  IdealPFdbkVariant=Disabled  SatFdbkVariant=Disabled  DerivativeFilterVariant=Disabled  NVariant=Disabled  NCopyVariant=Disabled_SignalSpec  FilterICVariant=Disabled  IntegratorICVariant=InternalICs  ExternalResetVariant=Disabled  TRSumVariant=Passthrough  SumFdbkVariant=Disabled  SumVariant=Sum_PI  TsampFilterVariant=InternalTs  TsampNgainVariant=Passthrough  TsampIntegralVariant=Disabled_SignalSpec  ExternalSaturationOutDataTypeStr=Inherit: Same as second input
  Sum1 : Sum  Inputs=-+|
  cv [-] : Outport
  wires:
  T [K]/1 -> Sum1/1
  Gain/1 -> PID Controller1/1
  Sum1/1 -> Gain/1
  PID Controller1/1 -> cv [-]/1
  T_ref [K]/1 -> Sum1/2

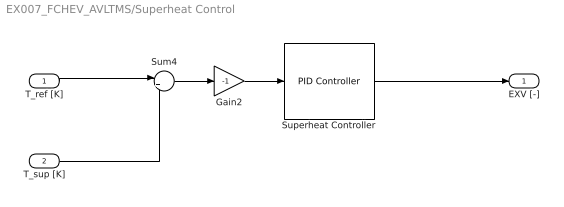
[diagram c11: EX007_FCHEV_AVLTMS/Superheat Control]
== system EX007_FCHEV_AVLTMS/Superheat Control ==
  T_ref [K] : Inport
  T_sup [K] : Inport  Port=2
  Gain2 : Gain  Gain=-1
  Sum4 : Sum  Inputs=|+-
  Superheat Controller : slpidlib/PID Controller  Controller=PI  Form=Parallel  TimeDomain=Continuous-time  UseExternalTs=off  SampleTime=-1  IntegratorMethod=Forward Euler  FilterMethod=Forward Euler  ControllerParametersSource=internal  P=1e-2  I=1e-2  UseKiTs=off  D=0  N=100  UseFilter=on  TunerSelectOption=Transfer Function Based (PID Tuner App)  InitialConditionSource=internal  InitialConditionForIntegrator=0.3  InitialConditionForFilter=0  DifferentiatorICPrevScaledInput=0  ExternalReset=none  TrackingMode=off  Kt=1  LimitOutput=on  SatLimitsSource=internal  UpperSaturationLimit=0.99  LowerSaturationLimit=0.01  LinearizeAsGain=on  AntiWindupMode=back-calculation  Kb=1  LimitIntegrator=off  UpperIntegratorSaturationLimit=inf  LowerIntegratorSaturationLimit=-inf  POutMin=[]  POutMax=[]  IOutMin=[]  IOutMax=[]  DOutMin=[]  DOutMax=[]  NOutMin=[]  NOutMax=[]  SumOutMin=[]  SumOutMax=[]  SaturationOutMin=[]  SaturationOutMax=[]  PParamMin=[]  PParamMax=[]  IParamMin=[]  IParamMax=[]  DParamMin=[]  DParamMax=[]  NParamMin=[]  NParamMax=[]  KbParamMin=[]  KbParamMax=[]  KtParamMin=[]  KtParamMax=[]  KbOutMin=[]  KbOutMax=[]  KtOutMin=[]  KtOutMax=[]  IntegratorOutMin=[]  IntegratorOutMax=[]  FilterOutMin=[]  FilterOutMax=[]  SumI1OutMin=[]  SumI1OutMax=[]  SumI2OutMin=[]  SumI2OutMax=[]  SumI3OutMin=[]  SumI3OutMax=[]  SumI4OutMin=[]  SumI4OutMax=[]  SumDOutMin=[]  SumDOutMax=[]  DifferentiatorOutMin=[]  DifferentiatorOutMax=[]  FilterDiffOutCoefMin=[]  FilterDiffOutCoefMax=[]  ReciprocalOutMin=[]  ReciprocalOutMax=[]  SumDenOutMin=[]  SumDenOutMax=[]  SumNumOutMin=[]  SumNumOutMax=[]  DivideOutMin=[]  DivideOutMax=[]  UdiffTsProdOutMin=[]  UdiffTsProdOutMax=[]  NTsProdOutMin=[]  NTsProdOutMax=[]  UintegralTsProdOutMin=[]  UintegralTsProdOutMax=[]  UngainTsProdOutMin=[]  UngainTsProdOutMax=[]  ClampingZeroOutDataTypeStr=Inherit: Inherit via back propagation  ClampingZeroOutMin=[]  ClampingZeroOutMax=[]  FilterDenConstantOutDataTypeStr=Inherit: Inherit via back propagation  FilterDenConstantOutMin=[]  FilterDenConstantOutMax=[]  PCopyOutDataTypeStr=Inherit: Inherit via back propagation  PCopyOutMin=[]  PCopyOutMax=[]  NCopyOutDataTypeStr=Inherit: Inherit via back propagation  NCopyOutMin=[]  NCopyOutMax=[]  IntegratorContinuousStateAttributes=''  IntegratorStateMustResolveToSignalObject=off  IntegratorRTWStateStorageClass=Auto  FilterContinuousStateAttributes=''  FilterStateMustResolveToSignalObject=off  FilterRTWStateStorageClass=Auto  ParallelPVariant=InternalParameters  IdealPVariant=Disabled  IVariant=InternalParameters  DVariant=Disabled  IntegratorVariant=Continuous  SatVariant=Enabled  AWVariant=BackCalculation  PCopyVariant=Disabled  TRVariant=Disabled  FdbkBlocksVariant=Forward  IdealPFdbkVariant=Disabled  SatFdbkVariant=Disabled  DerivativeFilterVariant=Disabled  NVariant=Disabled  NCopyVariant=Disabled_SignalSpec  FilterICVariant=Disabled  IntegratorICVariant=InternalICs  ExternalResetVariant=Disabled  TRSumVariant=Passthrough  SumFdbkVariant=Disabled  SumVariant=Sum_PI  TsampFilterVariant=InternalTs  TsampNgainVariant=Passthrough  TsampIntegralVariant=Disabled_SignalSpec  ExternalSaturationOutDataTypeStr=Inherit: Same as second input
  EXV [-] : Outport
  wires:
  Sum4/1 -> Gain2/1
  T_ref [K]/1 -> Sum4/1
  T_sup [K]/1 -> Sum4/2
  Gain2/1 -> Superheat Controller/1
  Superheat Controller/1 -> EXV [-]/1
